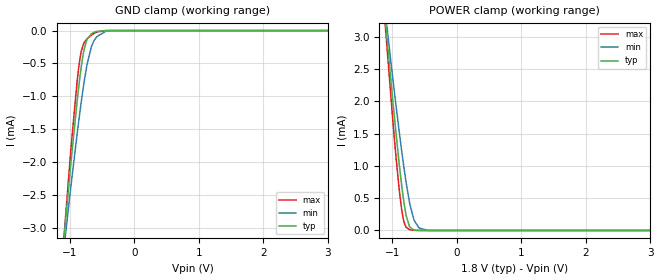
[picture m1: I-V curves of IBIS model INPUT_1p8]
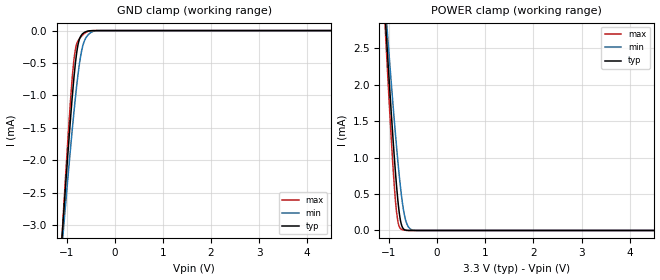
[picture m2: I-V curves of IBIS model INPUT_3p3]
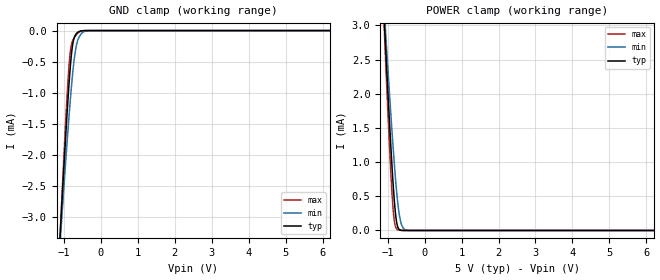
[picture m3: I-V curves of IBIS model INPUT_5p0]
|Texas Instruments Incorporated
|DACx3401 is a signle channel I2C interface, Buffered Voltage Output DAC
|DACx3401 comes in a Tiny 2*2 WSON package
[IBIS Ver] 4.1
[File name] dac11001.ibs
[File Rev] 1.0
[Date] 15/11/2019
[Source]
| Texas Instruments Incorporated.
| 12500 TI Blvd
| Dallas, TX -75243
[Notes] Revision History:
| Rev 1.0: 02/18/2019
| - Initial version of the model
| - Model generated from simulations in TISPICE/SPECTRE
| - C_comp although listed in numerical order of value are
| obtained from varying PVT conditions. For PVT conditions for
| each specific value refer the buffer description under
| respective [Model]. IBIS model user is responsible for using
| appropriate C_comp to simulate for Signal Integrity.
| - Warnings regarding combined Non-monotonicity of various models have been
| reviewed and considered minor and can be ignored.
| - Model names with a trailing _1p8 contain the model for 1.8V operation.
|   Model names with a trailing _3p3 contain the model for 3.3V operation.
|   Model names with a trailing _5p0 contain the model for 5.0V operation.
[Disclaimer]
| This model is designed as an aid for customers of Texas Instruments.
| TI and its licensors and suppliers make no warranties, either expressed
| or implied, with respect to this  model, including the warranties of
| merchantability or fitness for a particular purpose. The model is
| provided solely on an "as is" basis. The entire risk as to its quality
| and performance is with the customer.
| This model is subject to change without notice. Texas Instruments
| Incorporated is not responsible for updating this model.
[Copyright]
(C) Copyright 2018 Texas Instruments Incorporated.All rights reserved.
|  Component DAC11001 48-pin TQFP
|  Part # DAC11001
[Component]   DAC11001
[Manufacturer]  TI
[Package]   |48-pin TQFP
|   typ   min   max
R_pkg   0.05   0.04   0.06
L_pkg   1.0nH   0.8nH   1.2nH
C_pkg   0.2pF   0.16pF   0.24pF
[Pin]   signal_name   model_name   R_pin   L_pin   C_pin
1   NC   NC   NA   NA   NA
2   AGND   GND   NA   NA   NA
3   REFPF   NC   NA   NA   NA
4   REFPS   NC   NA   NA   NA
5   REFNF   NC   NA   NA   NA
6   REFNS   NC   NA   NA   NA
7   OUT   NC   NA   NA   NA
8   AGND_OUT   GND   NA   NA   NA
9   RFB   NC   NA   NA   NA
10   ROFS   NC   NA   NA   NA
11   RCM   NC   NA   NA   NA
12   NC   NC   NA   NA   NA
13   NC   NC   NA   NA   NA
14   AGND_TnH   GND   NA   NA   NA
15   NC   NC   NA   NA   NA
16   DGND   GND   NA   NA   NA
17   DGND   GND   NA   NA   NA
18   LDAC   INPUT   NA   NA   NA
19   ALARM   OPEN_SINK   NA   NA   NA
20   DGND   GND   NA   NA   NA
21   DGND   GND   NA   NA   NA
22   DGND   GND   NA   NA   NA
23   DGND   GND   NA   NA   NA
24   NC   NC   NA   NA   NA
25   NC   NC   NA   NA   NA
26   DGND   GND   NA   NA   NA
27   DVDD   POWER   NA   NA   NA
28   IOVDD   POWER   NA   NA   NA
29   NC   NC   NA   NA   NA
30   CLR   INPUT   NA   NA   NA
31   SCLK   INPUT   NA   NA   NA
32   SDIN   INPUT   NA   NA   NA
33   SYNC   INPUT   NA   NA   NA
34   SDO   OUTPUT   NA   NA   NA
35   AGND   GND   NA   NA   NA
36   NC   NC   NA   NA   NA
37   NC   NC   NA   NA   NA
38   AGND   GND   NA   NA   NA
39   AVDD   POWER   NA   NA   NA
40   AGND   GND   NA   NA   NA
41   AVDD   POWER   NA   NA   NA
42   AGND   GND   NA   NA   NA
43   AGND   GND   NA   NA   NA
44   VSS   GND   NA   NA   NA
45   VCC   POWER   NA   NA   NA
46   AGND   GND   NA   NA   NA
47   AGND   GND   NA   NA   NA
48   NC   NC   NA   NA   NA
|   Model Selectors
[Model Selector]   INPUT
INPUT_1p8   1.8V  digital Input
INPUT_3p3   3.3V  digital Input
INPUT_5p0   5.0V  digital Input
[Model Selector]   OUTPUT
OUTPUT_1p8   1.8V  digital Output
OUTPUT_3p3   3.3V  digital Output
OUTPUT_5p0   5.0V  digital Output
[Model Selector]   OPEN_SINK
OPEN_SINK_1p8   1.8V  digital Output_Open_Sink
OPEN_SINK_3p3   3.3V  digital Output_Open_Sink
OPEN_SINK_5p0   5.0V  digital Output_Open_Sink
| Models and submodels in the file (9): INPUT_1p8 (Input), INPUT_3p3 (Input), INPUT_5p0 (Input), OPEN_SINK_1p8 (Open_sink), OPEN_SINK_3p3 (Open_sink), OPEN_SINK_5p0 (Open_sink), OUTPUT_1p8 (3-state), OUTPUT_3p3 (3-state), OUTPUT_5p0 (3-state)
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|   INPUT_1p8 Model
[Model]   INPUT_1p8
Model_type   Input
Vinl = 0.54
Vinh = 1.26
|   typ   min   max
C_comp   0.42pF   0.405pF   0.424pF
[Voltage Range]   1.8   1.65   1.95
[Temperature Range]   25   125   -40
[Power Clamp Reference]   1.8   1.65   1.95
[GND Clamp Reference]   0   0   0
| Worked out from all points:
|   GND clamp passes 1 mA (typ) near -0.88 V on its own axis
|   POWER clamp passes 1 mA (typ) near -0.89 V on its own axis
[GND Clamp]
|   Voltage   I(typ)   I(min)   I(max)
-1.8V     -11.28mA   -9.914mA   -12.63mA
-1.157V   -3.894mA   -3.908mA   -3.98mA
-1.001V   -2.2mA     -2.523mA   -2.022mA
-968.4mV  -1.866mA   -2.246mA   -1.641mA
-887.4mV  -1.081mA   -1.579mA   -780.5uA
-833.4mV  -629.2uA   -1.164mA   -371.2uA
-774mV    -268.9uA   -755.5uA   -177.8uA
-730.8mV  -130.7uA   -507.1uA   -124.6uA
-660.6mV  -46.3uA    -232.1uA   -65.84uA
-579.6mV  -12.67uA   -91.77uA   -20.72uA
-374.4mV  -55.14nA   -1.954uA   -54.45nA
3.6V      0A         0A         0A
[POWER Clamp]
|   Voltage   I(typ)   I(min)   I(max)
-1.8V     11.19mA    9.813mA    12.51mA
-1.152V   3.733mA    3.762mA    3.717mA
-1.001V   2.098mA    2.427mA    1.808mA
-941.4mV  1.493mA    1.925mA    1.125mA
-855mV    700.9uA    1.235mA    325uA
-817.2mV  418.1uA    956.6uA    127.3uA
-784.8mV  230.3uA    736.2uA    49.78uA
-736.2mV  67.63uA    449.8uA    13.71uA
-666mV    7.115uA    169.5uA    2.431uA
-585mV    495.9nA    37.8uA     250.2nA
-444.6mV  1.371nA    1.045uA    0A
3.6V      0A         0A         0A
|   INPUT_3p3 Model
[Model]   INPUT_3p3
Model_type   Input
Vinl = 0.99
Vinh = 2.31
|   typ   min   max
C_comp   0.397pF   0.394pF   0.407pF
[Voltage Range]   3.3   3   3.6
[Temperature Range]   25   125   -40
[Power Clamp Reference]   3.3   3   3.6
[GND Clamp Reference]   0   0   0
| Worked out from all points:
|   GND clamp passes 1 mA (typ) near -0.88 V on its own axis
|   POWER clamp passes 1 mA (typ) near -0.89 V on its own axis
[GND Clamp]
|   Voltage   I(typ)   I(min)   I(max)
-3.3V     -29.05mA   -24.39mA   -33.52mA
-1.142V   -3.721mA   -3.768mA   -3.78mA
-1.073V   -2.963mA   -3.149mA   -2.901mA
-1.063V   -2.856mA   -3.062mA   -2.778mA
-924mV    -1.424mA   -1.875mA   -1.147mA
-844.8mV  -717.1uA   -1.249mA   -439.5uA
-795.3mV  -376.4uA   -894.8uA   -221.6uA
-745.8mV  -167.6uA   -587.4uA   -140.3uA
-676.5mV  -57.89uA   -279.3uA   -77.67uA
-597.3mV  -17.43uA   -112.1uA   -28.12uA
-369.6mV  -42.8nA    -1.709uA   -41.07nA
6.6V      0A         0A         0A
[POWER Clamp]
|   Voltage   I(typ)   I(min)   I(max)
-3.3V     28.95mA    24.28mA    33.42mA
-1.092V   3.076mA    3.228mA    2.946mA
-1.073V   2.861mA    3.052mA    2.694mA
-1.063V   2.754mA    2.965mA    2.569mA
-1.013V   2.227mA    2.533mA    1.956mA
-924mV    1.323mA    1.781mA    939.5uA
-864.6mV  780.8uA    1.308mA    394.2uA
-805.2mV  341.7uA    872.7uA    90.27uA
-726mV    49.93uA    398.3uA    10.69uA
-627mV    1.945uA    86.31uA    855nA
-448.8mV  12.01nA    1.173uA    0A
6.6V      0A         0A         0A
|   INPUT_5p0 Model
[Model]   INPUT_5p0
Model_type   Input
Vinl = 1.5
Vinh = 3.5
|   typ   min   max
C_comp   0.376pF   0.358pF   0.389pF
[Voltage Range]   5   4.5   5.5
[Temperature Range]   25   125   -40
[Power Clamp Reference]   5   4.5   5.5
[GND Clamp Reference]   0   0   0
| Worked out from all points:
|   GND clamp passes 1 mA (typ) near -0.88 V on its own axis
|   POWER clamp passes 1 mA (typ) near -0.89 V on its own axis
[GND Clamp]
|   Voltage   I(typ)   I(min)   I(max)
-5V       -49.36mA   -40.97mA   -57.39mA
-1.115V   -3.426mA   -3.527mA   -3.438mA
-1.085V   -3.098mA   -3.26mA    -3.058mA
-920mV    -1.386mA   -1.842mA   -1.105mA
-875mV    -969.9uA   -1.481mA   -669.4uA
-830mV    -603.9uA   -1.14mA    -353uA
-770mV    -251.7uA   -730.4uA   -171.5uA
-710mV    -94.12uA   -407.7uA   -105.3uA
-635mV    -31.96uA   -172.2uA   -48.63uA
-545mV    -6.324uA   -60.92uA   -10.38uA
-305mV    0A         -264.8nA   0A
10V       0A         0A         0A
[POWER Clamp]
|   Voltage   I(typ)   I(min)   I(max)
-5V       49.26mA    40.86mA    57.29mA
-1.1V     3.16mA     3.296mA    3.044mA
-1.04V    2.512mA    2.767mA    2.287mA
-950mV    1.579mA    1.996mA    1.22mA
-875mV    870.3uA    1.389mA    476.5uA
-815mV    403.5uA    941uA      119.7uA
-770mV    165.5uA    642.5uA    32.8uA
-725mV    48.43uA    393.4uA    10.43uA
-680mV    11.34uA    211.2uA    3.462uA
-620mV    1.541uA    75.78uA    698.6nA
-410mV    0A         381.1nA    0A
10V       0A         0A         0A
